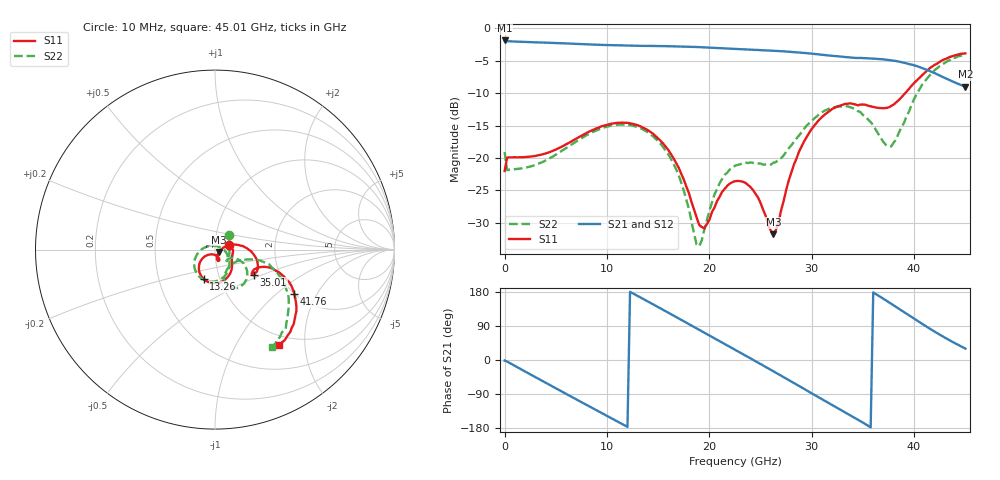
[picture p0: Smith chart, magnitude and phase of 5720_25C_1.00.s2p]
! Device:  ADRF5720
! Description: 0.5dB LSB GaAs MMIC 6-bit Digital Attenuator
! Frequency:  0.000009 -  40 GHz
! Ports:
!	RF1	= Port 1
!	RF2	= Port 2
! Vdd:  3.3 Volt
! Vss:  -3.3 Volt
! Control:  0/3.3 Volt
! State:  1.00 dB attenuation
! Data:  The device was measured using G-S-G Probes on a matrix board.
!  Data was collected using an calibrated 4 port network analyzer.
!  The reference plane for this measurement is at the launchers.
! Note:  Analog Devices supplies this data as a sample of measured data
!  for this product.  Your particular data for this product may vary.
!  Data was taken at 25 degrees C.
!  Analog Devices reserves the right to change this data at anytime.
# GHZ S DB R 45.0
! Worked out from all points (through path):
!   181 points, 10 MHz to 45.01 GHz, reference 45 ohm
!   highest |S21| = -1.86 dB at 10 MHz (marker M1); lowest = -9.0 dB at 45.01 GHz (marker M2)
!   group delay of S21, straight-line fit = 42.4 ps
!   lowest |S11| = -31.8 dB at 26.26 GHz (marker M3), VSWR 1.05, Z = 47 - j1.31 ohm
!   |S11| at or under -10 dB: start of sweep to 39.13 GHz
!   |S22| runs from -33.6 to -4.0 dB; largest |S21 - S12| = 0.00098
!   S11 on the Smith chart (normalised r, x): 10 MHz: 1.16, +0.05; 13.26 GHz: 0.84, -0.28; 35.01 GHz: 1.48, -0.44; 41.76 GHz: 1.99, -1.33; 45.01 GHz: 0.84, -1.53
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0.01  -22.02 16.9  -1.86 -1.5  -1.86 -1.5  -19.11 45.4
0.26  -19.95 -0.8  -1.98 -4.2  -1.98 -4.2  -21.91 -0.7
2.26  -19.84 -18.8  -2.10 -34.1  -2.10 -34.1  -21.44 -20.4
4.26  -19.19 -31.4  -2.21 -63.6  -2.21 -63.6  -20.20 -34.9
7.76  -16.36 -54.5  -2.44 -114.9  -2.43 -114.8  -16.73 -62.5
10.76  -14.64 -83.7  -2.61 -158.4  -2.61 -158.4  -14.93 -94.4
13.26  -15.12 -111.2  -2.69 165.3  -2.69 165.3  -15.42 -125.2
15.26  -17.39 -131.6  -2.73 135.8  -2.73 135.9  -17.88 -152.6
17.01  -21.51 -145.1  -2.78 109.8  -2.78 109.8  -22.71 178.1
19.01  -30.36 -121.1  -2.89 79.7  -2.89 79.7  -33.64 75.2
21.01  -25.99 -65.8  -3.04 49.6  -3.04 49.6  -23.90 -13.8
22.76  -23.56 -72.0  -3.18 23.3  -3.18 23.3  -21.08 -35.6
24.51  -25.53 -77.4  -3.32 -3.1  -3.32 -3.0  -20.88 -44.6
26.26  -31.81 -32.8  -3.45 -29.8  -3.45 -29.8  -20.75 -34.0
28.26  -21.05 16.5  -3.65 -60.8  -3.65 -60.7  -17.54 -23.1
30.26  -15.00 2.5  -3.94 -91.9  -3.94 -91.9  -13.89 -30.8
32.51  -12.07 -17.6  -4.29 -126.6  -4.29 -126.5  -12.06 -49.8
35.01  -11.75 -32.7  -4.58 -165.4  -4.58 -165.3  -13.38 -70.6
37.76  -11.97 -24.7  -4.92 148.6  -4.93 148.7  -18.23 -40.0
39.76  -8.85 -19.3  -5.59 113.5  -5.59 113.5  -11.77 -13.6
41.76  -5.89 -29.3  -6.74 79.0  -6.74 79.0  -6.88 -28.9
45.01  -3.85 -56.1  -8.99 30.0  -8.99 30.1  -4.03 -59.4
